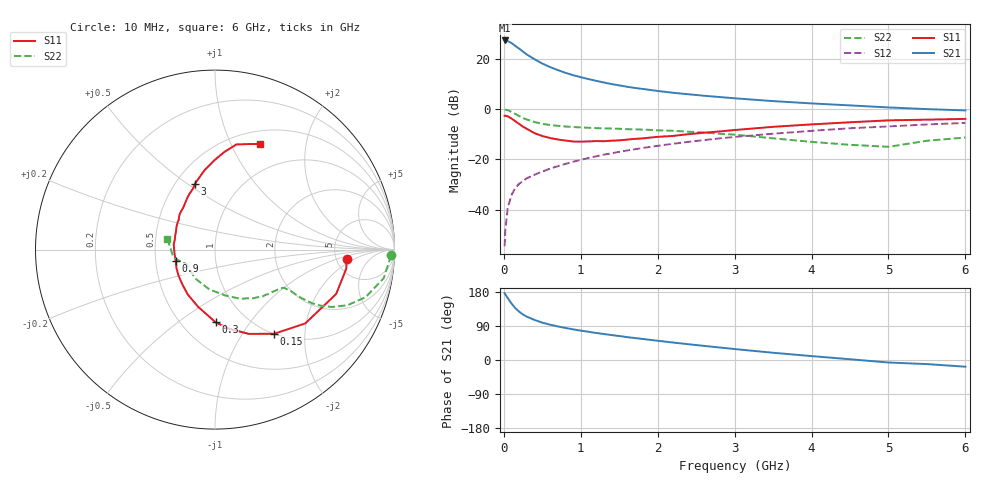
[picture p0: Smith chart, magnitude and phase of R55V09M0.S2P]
! SIEMENS Small Signal Semiconductors
! BFR183
! Si NPN RF Bipolar Junction Transistor in SOT23
! VCE = 5 V  IC = 9 mA
! Common Emitter S-Parameters:  May  1996
# GHz  S  MA  R  50
!  f  S11  S21  S12  S22
! GHz  MAG  ANG  MAG  ANG  MAG  ANG  MAG  ANG
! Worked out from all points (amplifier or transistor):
!   36 points, 10 MHz to 6 GHz, reference 50 ohm
!   highest |S21| = 27.3 dB at 10 MHz (marker M1)
!   |S21| within 3 dB of that: start of sweep to 187.4 MHz
!   unconditionally stable (mu >= 1): 822.7 MHz to 2.537 GHz
!   at 250 MHz: K = 0.58, MSG = 25.6 dB, |S12| = -28.5 dB
!   at 1.4 GHz: K = 1.05, MAG = 12.3 dB, |S12| = -17.5 dB
!   at 6 GHz: K = 0.89, MSG = 2.5 dB, |S12| = -5.5 dB
!   S11 on the Smith chart (normalised r, x): 10 MHz: 6.24, -1.47; 150 MHz: 1.00, -1.40; 300 MHz: 0.72, -0.70; 900 MHz: 0.64, -0.08; 3 GHz: 0.62, +0.54; 6 GHz: 0.65, +1.29
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0.01  0.7368 -4.2  23.06 176.5  0.0019 83.6  0.9815 -1.9
0.02  0.7388 -8.3  22.81 172.9  0.0041 77.7  0.9725 -3.9
0.05  0.719 -20.1  22.37 163.5  0.0108 79.4  0.9534 -9.6
0.1  0.6496 -39.3  20.5 149.0  0.0198 71.9  0.8804 -17.5
0.15  0.5731 -54.9  17.93 136.7  0.0274 67.3  0.8004 -22.8
0.2  0.5062 -68.1  15.82 127.3  0.033 64.3  0.727 -26.1
0.25  0.4473 -80.1  13.79 119.9  0.0377 62.6  0.6649 -28.0
0.3  0.4051 -89.5  12.12 114.2  0.0424 62.1  0.6198 -28.9
0.4  0.3321 -106.5  9.748 105.7  0.0499 61.9  0.5534 -29.3
0.5  0.2927 -121.1  8.029 98.6  0.0575 62.8  0.5092 -29.0
0.6  0.2668 -132.7  6.851 93.3  0.0656 63.4  0.4834 -28.7
0.7  0.2495 -144.5  5.968 88.7  0.0735 64.1  0.466 -28.8
0.9  0.2273 -164.0  4.724 80.9  0.0901 64.3  0.4409 -28.9
1.1  0.228 179.2  3.947 74.5  0.1071 64.7  0.4261 -30.4
1.3  0.2305 166.0  3.373 68.6  0.1246 64.0  0.4147 -32.0
1.6  0.2478 150.3  2.778 60.4  0.1506 62.4  0.4003 -35.6
2.2  0.2936 127.0  2.109 46.1  0.205 58.1  0.3711 -44.7
3  0.3843 106.8  1.64 28.9  0.2804 50.0  0.3109 -62.0
3.5  0.445 97.7  1.441 19.1  0.3245 44.0  0.2631 -77.0
4.5  0.5477 84.4  1.185 2.0  0.4166 31.9  0.1955 -124.3
5.5  0.6173 72.3  1 -10.8  0.4953 20.1  0.2352 -169.0
6  0.6393 67.0  0.941 -17.7  0.5324 12.4  0.2727 167.0
